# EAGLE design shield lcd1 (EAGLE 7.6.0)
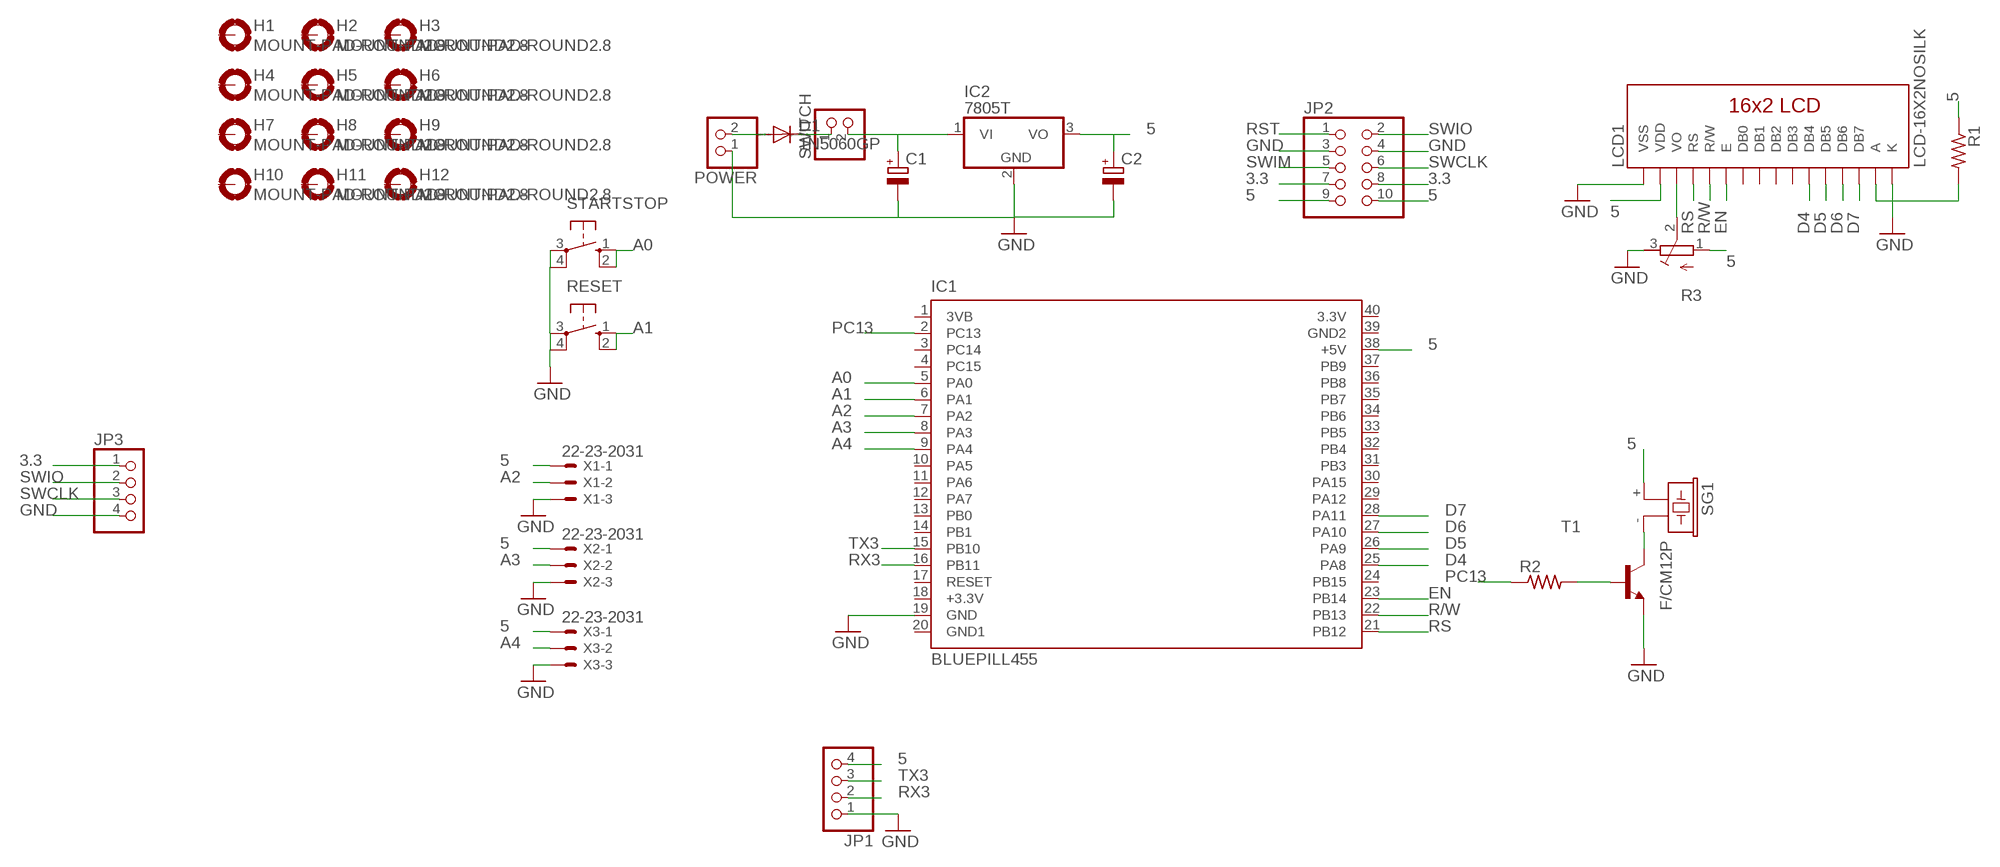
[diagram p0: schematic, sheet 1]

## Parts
C1  CPOL-EUE2.5-7  [E2,5-7]
C2  CPOL-EUE2.5-6  [E2,5-6]
D1  1N5060GP  [DO15-12]
H1  MOUNT-PAD-ROUND2.8  [2,8-PAD]
H2  MOUNT-PAD-ROUND2.8  [2,8-PAD]
H3  MOUNT-PAD-ROUND2.8  [2,8-PAD]
H4  MOUNT-PAD-ROUND2.8  [2,8-PAD]
H5  MOUNT-PAD-ROUND2.8  [2,8-PAD]
H6  MOUNT-PAD-ROUND2.8  [2,8-PAD]
H7  MOUNT-PAD-ROUND2.8  [2,8-PAD]
H8  MOUNT-PAD-ROUND2.8  [2,8-PAD]
H9  MOUNT-PAD-ROUND2.8  [2,8-PAD]
H10  MOUNT-PAD-ROUND2.8  [2,8-PAD]
H11  MOUNT-PAD-ROUND2.8  [2,8-PAD]
H12  MOUNT-PAD-ROUND2.8  [2,8-PAD]
IC1  BLUEPILL455  [DIL40]
IC2  7805T  [TO220H]
JP1  PINHD-1X4  [1X04]
JP2  PINHD-2X5  [2X05]
JP3  PINHD-1X4  [1X04]
LCD1  LCD-16X2NOSILK  [LCD-16X2_NOSILK]
POWER  PINHD-1X2  [1X02]
R1  R-US_0207/10  [0207/10]
R2  R-US_M0805  [M0805]
R3  R-TRIMM3339P  [RTRIM3339P]
RESET  40-XX  [B3F-40XX]
SG1  F/CM12P  [F/CM12P]
STARTSTOP  40-XX  [B3F-40XX]
SWITCH  PINHD-1X2  [1X02]
T1  BF820-NPN-SOT23-BEC  [SOT23-BEC]
X1  22-23-2031  [22-23-2031]
X2  22-23-2031  [22-23-2031]
X3  22-23-2031  [22-23-2031]

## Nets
3.3: JP2.7 JP2.8 JP3.1
5: C2.+ IC1.38(+5V) IC2.3(VO) JP1.4 JP2.9 JP2.10 LCD1.2(VDD) R1.1 R3.1(A) SG1.+ X1.1 X2.1 X3.1
A0: IC1.5(PA0) STARTSTOP.1(S) STARTSTOP.2(S1)
A1: IC1.6(PA1) RESET.1(S) RESET.2(S1)
A2: IC1.7(PA2) X1.2
A3: IC1.8(PA3) X2.2
A4: IC1.9(PA4) X3.2
D4: IC1.25(PA8) LCD1.11(DB4)
D5: IC1.26(PA9) LCD1.12(DB5)
D6: IC1.27(PA10) LCD1.13(DB6)
D7: IC1.28(PA11) LCD1.14(DB7)
EN: IC1.23(PB14) LCD1.6(E)
GND: C1.- C2.- IC1.19(GND) IC2.2(GND) JP1.1 JP2.3 JP2.4 JP3.4 LCD1.1(VSS) LCD1.16(K) POWER.1 R3.3(E) RESET.3(P) RESET.4(P1) STARTSTOP.3(P) STARTSTOP.4(P1) T1.E X1.3 X2.3 X3.3
N$1: LCD1.15(A) R1.2
N$2: R2.2 T1.B
N$9: C1.+ IC2.1(VI) SWITCH.2
N$10: SG1.- T1.C
N$12: LCD1.3(VO) R3.2(S)
N$13: D1.C SWITCH.1
N$14: D1.A POWER.2
PC13: IC1.2(PC13) R2.1
R/W: IC1.22(PB13) LCD1.5(R/W)
RS: IC1.21(PB12) LCD1.4(RS)
RST: JP2.1
RX3: IC1.16(PB11) JP1.2
SWCLK: JP2.6 JP3.3
SWIM: JP2.5
SWIO: JP2.2 JP3.2
TX3: IC1.15(PB10) JP1.3
Unconnected: H1.B2,8(MOUNT) H2.B2,8(MOUNT) H3.B2,8(MOUNT) H4.B2,8(MOUNT) H5.B2,8(MOUNT) H6.B2,8(MOUNT) H7.B2,8(MOUNT) H8.B2,8(MOUNT) H9.B2,8(MOUNT) H10.B2,8(MOUNT) H11.B2,8(MOUNT) H12.B2,8(MOUNT) IC1.1(3VB) IC1.3(PC14) IC1.4(PC15) IC1.10(PA5) IC1.13(PB0) IC1.14(PB1) IC1.17(RESET) IC1.18(+3.3V) IC1.20(GND1) IC1.24(PB15) IC1.29(PA12) IC1.30(PA15) IC1.33(PB5) IC1.34(PB6) IC1.35(PB7) IC1.36(PB8) IC1.37(PB9) IC1.39(GND2) IC1.40(3.3V) LCD1.7(DB0) LCD1.8(DB1) LCD1.9(DB2) LCD1.10(DB3)

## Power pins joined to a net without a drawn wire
PA6: IC1.11(PA6)
PA7: IC1.12(PA7)
PB3: IC1.31(PB3)
PB4: IC1.32(PB4)

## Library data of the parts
C1 C2 = resistor:CPOL-EU: POLARIZED CAPACITOR, European symbol
D1 = diode:1N5060GP: DIODE
H1-H12 = holes:MOUNT-PAD-ROUND: MOUNTING PAD, round
IC1 = STM32BluePill:BLUEPILL: BluePill STM32F108T6 Dev Board Source: http://www.stm32duino.com; 0: x; MF: BluePill; MPN: BluePill; X: 0
IC2 = linear:78*: Positive VOLTAGE REGULATOR Source: http://cache.national.com/ds/LM/LM78L05.pdf http://www.fairchildsemi.com/ds/LM/LM7805.pdf
JP1 JP3 = pinhead:PINHD-1X4: PIN HEADER
JP2 = pinhead:PINHD-2X5: PIN HEADER
LCD1 = SparkFun-Displays:LCD-16X2: Standard text-only 16x2 parallel input LCD Basic 16 character by 2 line display. Typically utilizes the extremely common HD44780 parallel interface chipset SparkFun Products: Basic 16x2 Green Basic 8x2 Green; SF_ID: LCD-00255
POWER SWITCH = pinhead:PINHD-1X2: PIN HEADER
R1 R2 = resistor:R-US_: RESISTOR, American symbol
R3 = resistor:R-TRIMM: Trimm resistor
RESET STARTSTOP = switch-omron:40-XX: OMRON SWITCH; MF: OMRON COMPONENTS USA; MPN: B3F-4000; OC_FARNELL: 176434; OC_NEWARK: 36K3105
SG1 = buzzer:F/CM12P: BUZZER; OC_FARNELL: unknown; OC_NEWARK: unknown
T1 = transistor:*-NPN-: NPN Transistror BF959 corrected 2008.03.06
X1-X3 = con-molex:22-23-2031: .100" (2.54mm) Center Header - 3 Pin; MF: MOLEX; MPN: 22-23-2031; OC_FARNELL: 1462950; OC_NEWARK: 30C0862

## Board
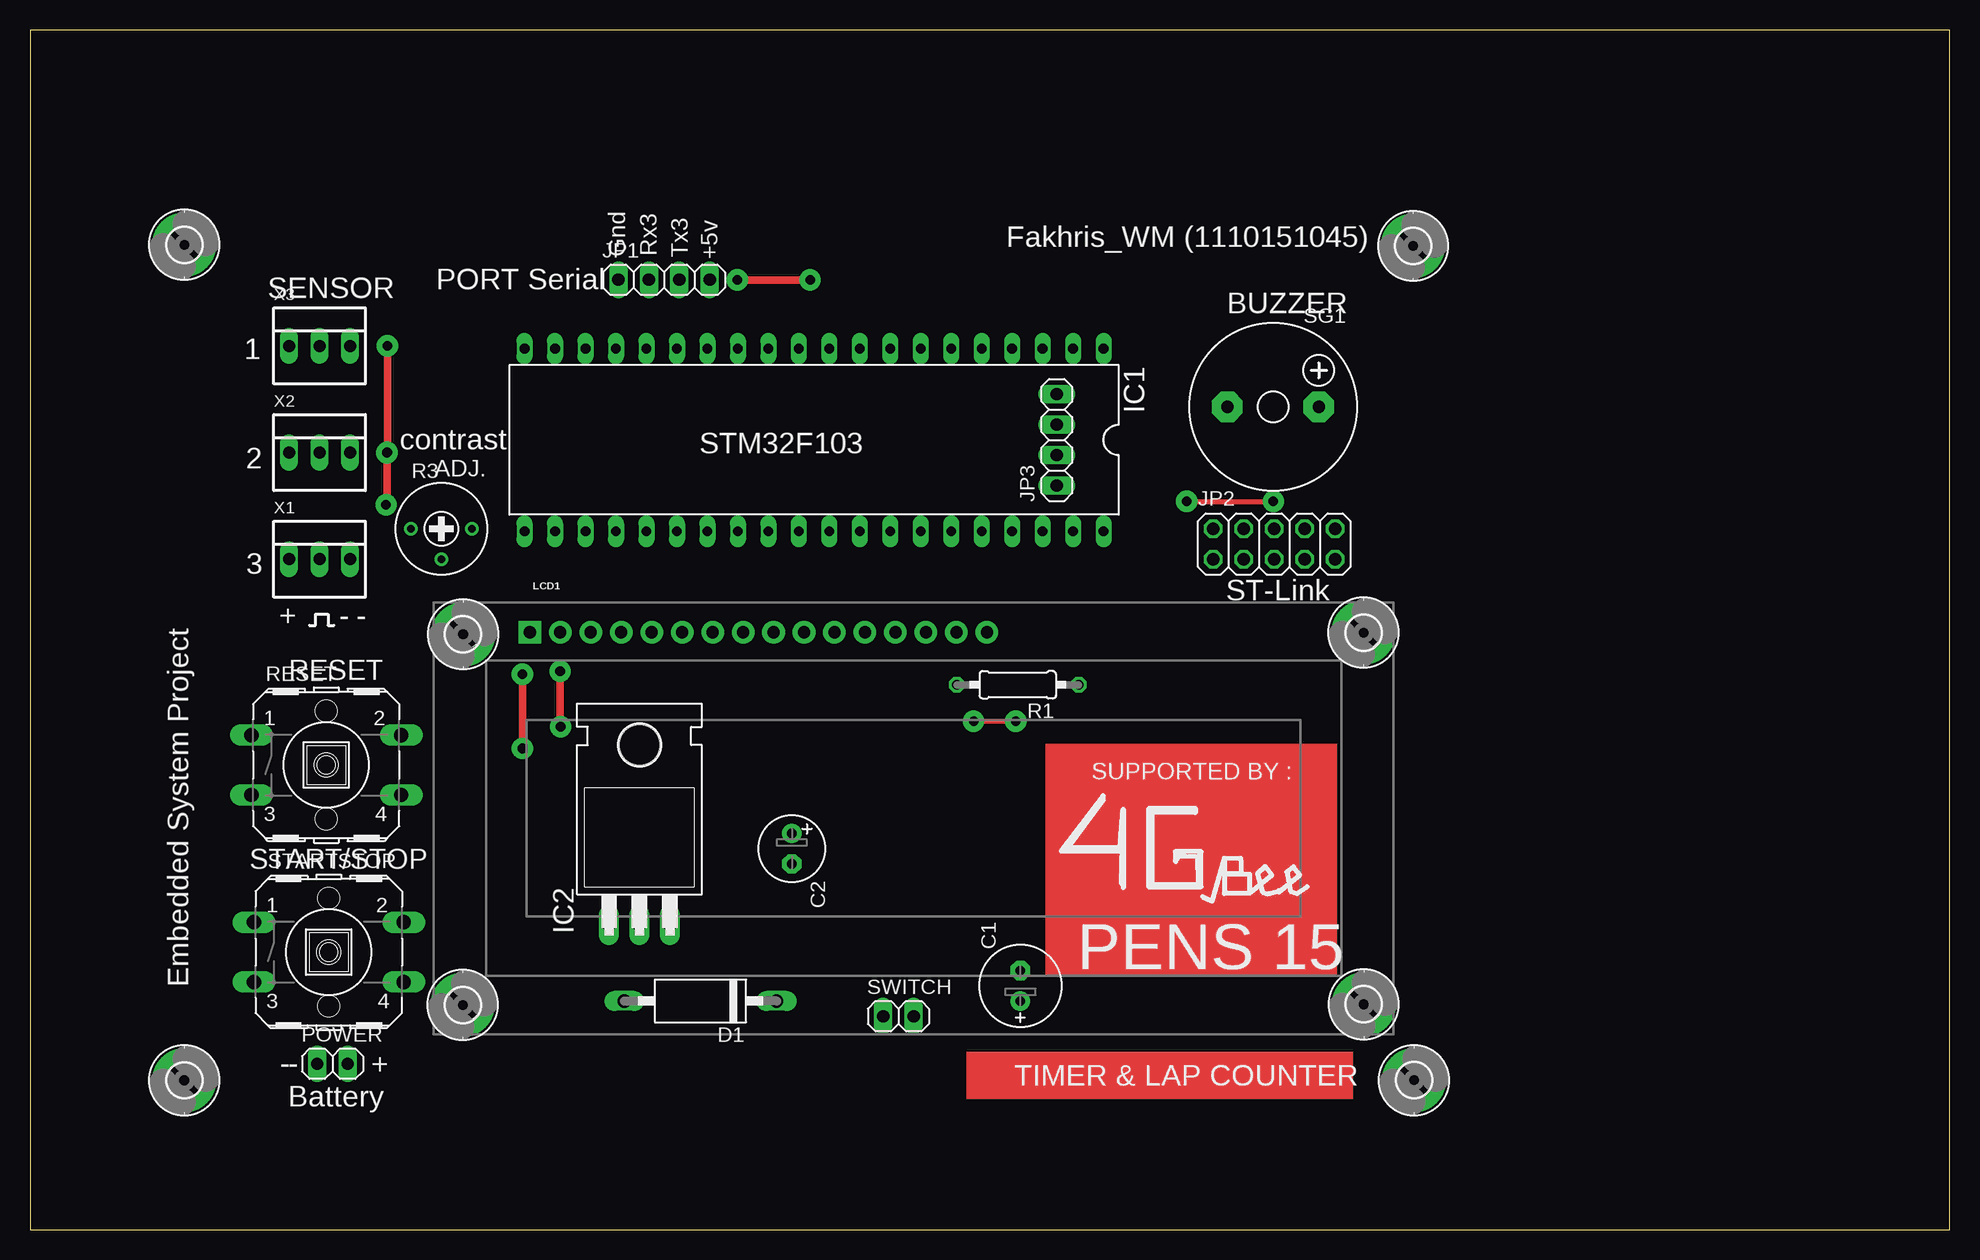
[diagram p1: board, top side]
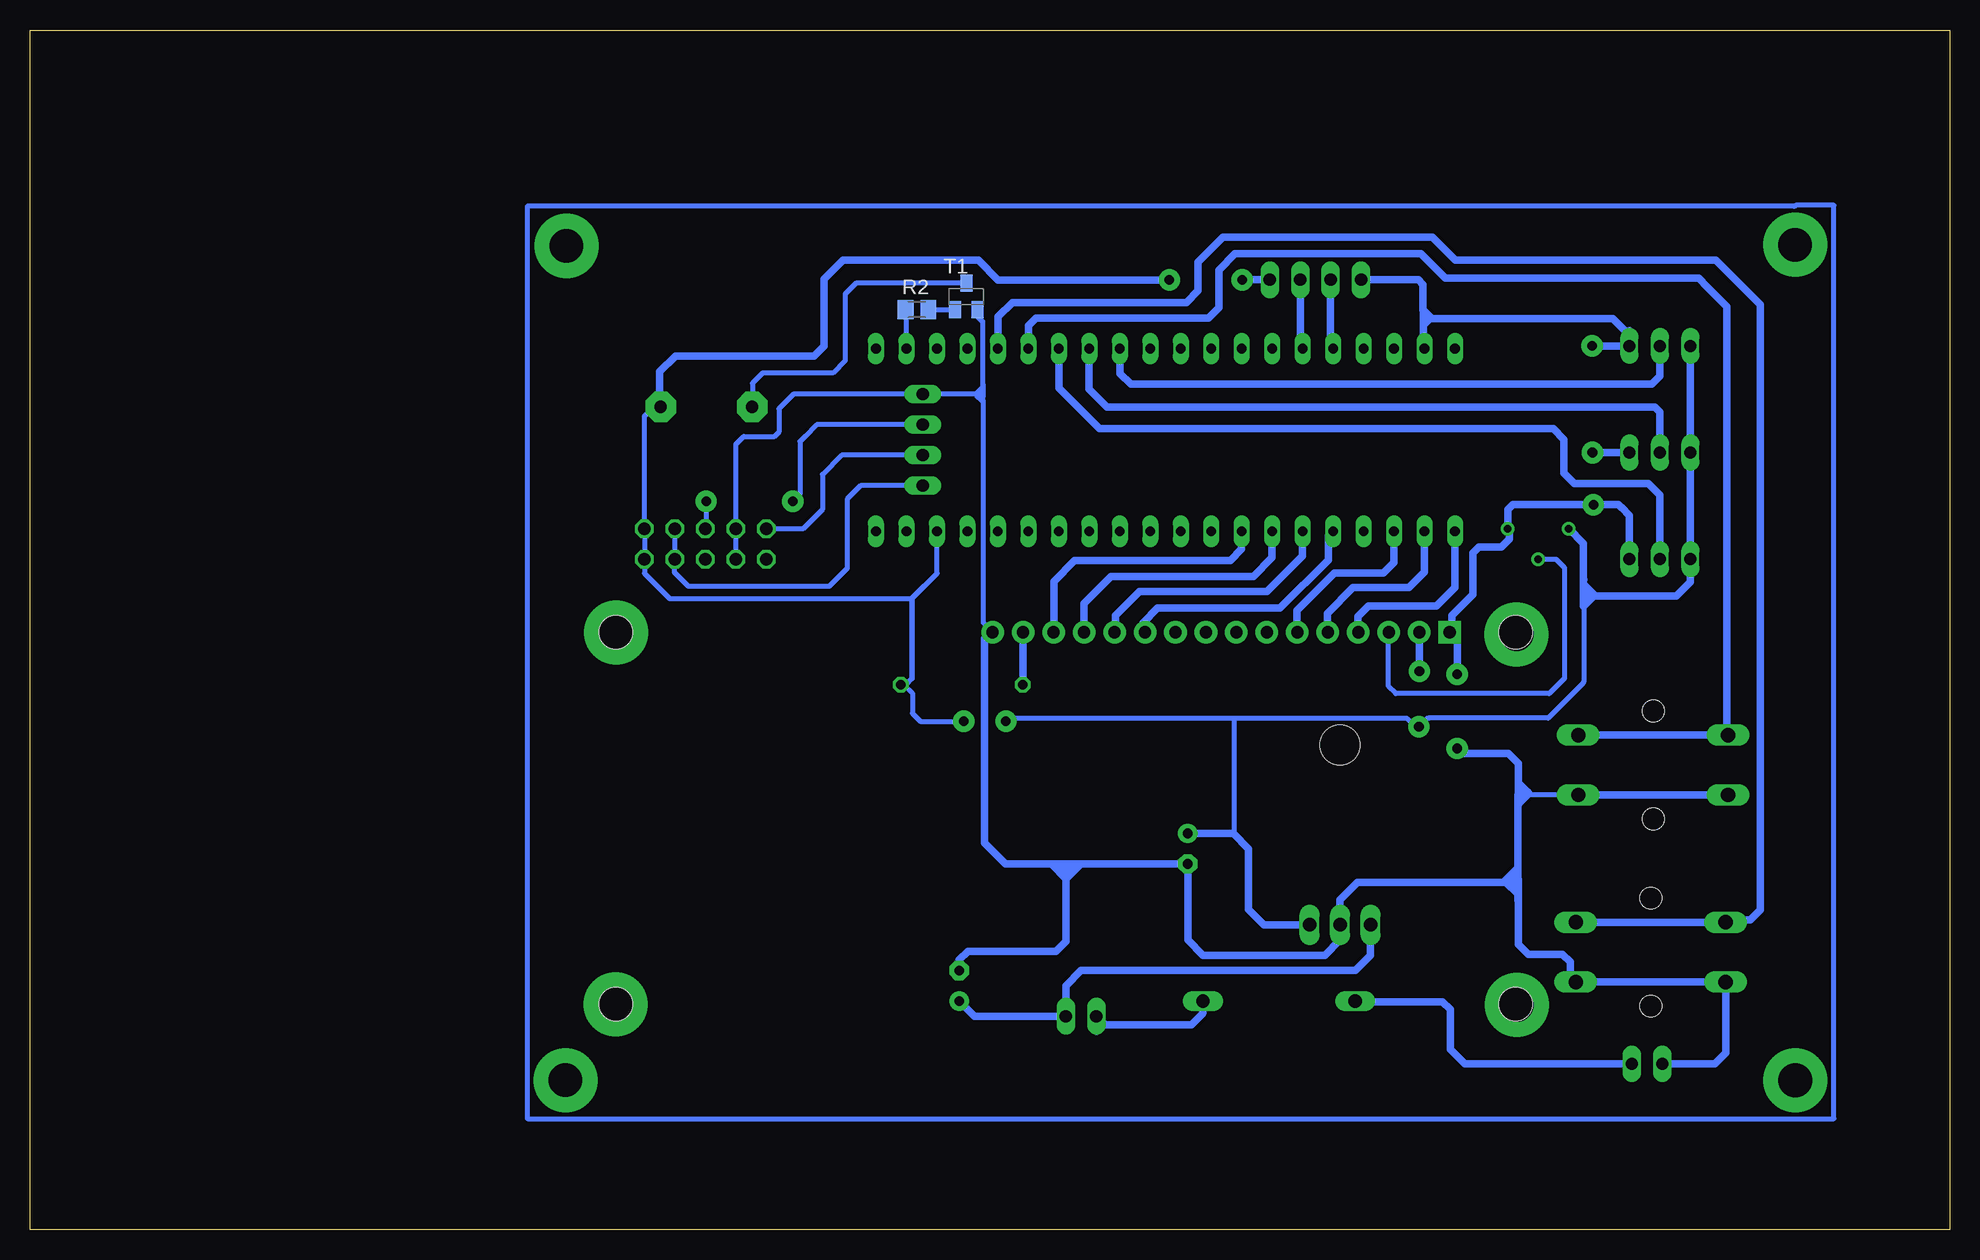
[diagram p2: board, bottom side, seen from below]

Size 160 x 100 mm. Coordinates in mm from the lower left corner, seen from the top.
Outline: 0,0 160,0 160,100 0,100 0,0
Copper layers (1*16): Top 0.035mm / dielectric 1.5mm / Bottom 0.035mm
Design rules "default": minimum track width 10mil, minimum drill 24mil, track to track 8mil, track to pad 8mil, pad to pad 8mil, via to via 8mil, smd to smd 8mil, copper to edge 40mil, drill to drill 8mil, minimum pad ring 10mil, minimum via ring 8mil, stop-mask expansion 4mil, vias tented up to drill 0mil, thermal gap 10mil

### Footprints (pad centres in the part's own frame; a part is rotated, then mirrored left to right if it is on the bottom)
E2,5-7 = drill 0.813 pad 1.6: + -1.27,0 | drill 0.813 pad 1.6 octagon: - 1.27,0
E2,5-6 = drill 0.813 pad 1.6: + -1.27,0 | drill 0.813 pad 1.6 octagon: - 1.27,0
DO15-12 = drill 1.118 long: A 6.35,0; C -6.35,0
2,8-PAD = drill 2.8 pad 5.334: B2,8 0,0
DIL40 = drill 0.813 long: 1 -24.13,-7.62; 2 -21.59,-7.62; 3 -19.05,-7.62; 4 -16.51,-7.62; 5 -13.97,-7.62; 6 -11.43,-7.62; 7 -8.89,-7.62; 8 -6.35,-7.62; 9 -3.81,-7.62; 10 -1.27,-7.62; 11 1.27,-7.62; 12 3.81,-7.62; 13 6.35,-7.62; 14 8.89,-7.62; 15 11.43,-7.62; 16 13.97,-7.62; 17 16.51,-7.62; 18 19.05,-7.62; 19 21.59,-7.62; 20 24.13,-7.62; 21 24.13,7.62; 22 21.59,7.62; 23 19.05,7.62; 24 16.51,7.62; 25 13.97,7.62; 26 11.43,7.62; 27 8.89,7.62; 28 6.35,7.62; 29 3.81,7.62; 30 1.27,7.62; 31 -1.27,7.62; 32 -3.81,7.62; 33 -6.35,7.62; 34 -8.89,7.62; 35 -11.43,7.62; 36 -13.97,7.62; 37 -16.51,7.62; 38 -19.05,7.62; 39 -21.59,7.62; 40 -24.13,7.62
TO220H = drill 1.118 long: 1 -2.54,-10.16; 2 0,-10.16; 3 2.54,-10.16 | hole 3.302: 0,4.826
1X04 = drill 1.016 long: 1 -3.81,0; 2 -1.27,0; 3 1.27,0; 4 3.81,0
2X05 = drill 1.016 octagon: 1 -5.08,-1.27; 2 -5.08,1.27; 3 -2.54,-1.27; 4 -2.54,1.27; 5 0,-1.27; 6 0,1.27; 7 2.54,-1.27; 8 2.54,1.27; 9 5.08,-1.27; 10 5.08,1.27
LCD-16X2_NOSILK = drill 1.016 pad 1.88 square: 1 -32,15.5 | drill 1.016 pad 1.88: 2 -29.46,15.5; 3 -26.92,15.5; 4 -24.38,15.5; 5 -21.84,15.5; 6 -19.3,15.5; 7 -16.76,15.5; 8 -14.22,15.5; 9 -11.68,15.5; 10 -9.14,15.5; 11 -6.6,15.5; 12 -4.06,15.5; 13 -1.52,15.5; 14 1.02,15.5; 15 3.56,15.5; 16 6.1,15.5 | hole 2.8: -37.5,15.5; -37.5,-15.5; 37.5,15.5; 37.5,-15.5
1X02 = drill 1.016 long: 1 -1.27,0; 2 1.27,0
0207/10 = drill 0.813 octagon: 1 -5.08,0; 2 5.08,0
M0805 = smd 1.3 x 1.6: 1 -0.95,0; 2 0.95,0
RTRIM3339P = drill 0.61: 1 -2.54,0; 2 0,-2.54; 3 2.54,0
B3F-40XX = drill 1.194 long: 1 -6.248,2.489; 2 6.248,2.489; 3 -6.248,-2.489; 4 6.248,-2.489 | hole 1.803: 0,-4.496; 0,4.496
F/CM12P = drill 1.016 pad 2.54 octagon: + 3.81,0; - -3.81,0
SOT23-BEC = smd 1 x 1.4: B -0.95,-1.1; C 0,1.1; E 0.95,-1.1
22-23-2031 = drill 1 long: 1 -2.54,0; 2 0,0; 3 2.54,0

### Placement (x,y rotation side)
C1  82.55,20.32 90 top
C2  63.5,31.75 270 top
D1  55.88,19.05 180 top
H1  111.16,49.76 0 top
H2  36.1,49.62 0 top
H3  36.08,18.72 0 top
H4  111.17,18.78 0 top
H5  115.36,12.45 0 top
H6  115.29,82 0 top
H7  12.87,82.09 0 top
H8  12.86,12.44 0 top
H9  not placed on the board
H10  not placed on the board
H11  not placed on the board
H12  not placed on the board
IC1  65.35,65.82 180 top
IC2  50.8,35.56 0 top
JP1  52.85,79.18 0 top
JP2  103.71,57.15 0 top
JP3  85.59,65.83 90 top
LCD1  73.66,34.29 0 top
POWER  25.21,13.82 0 top
R1  82.34,45.41 180 top
R2  86.07,76.69 0 bottom
R3  34.29,58.42 0 top
RESET  24.69,38.72 0 top
SG1  103.62,68.58 0 top
STARTSTOP  24.9,23.13 0 top
SWITCH  72.39,17.78 0 top
T1  81.96,77.78 0 bottom
X1  24.13,55.88 0 top
X2  24.13,64.77 0 top
X3  24.13,73.66 0 top

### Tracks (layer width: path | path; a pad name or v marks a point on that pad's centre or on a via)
3.3
  Bottom 0.406: JP3.1 90.75,62.02 91.89,60.88 91.89,55.11 93.38,53.62 105.11,53.62 106.28,54.78 106.28,55.85 JP2.7 | 106.29,55.83 JP2.7 | JP2.7 JP2.8
5  (via drill 0.8 pad 1.78)
  Top 0.406: v82.17,42.36 78.66,42.36 v78.65,42.37
  Top 0.61: v44.19,46.54 44.19,42.42 v44.23,41.93 | v58.95,79.17 v65.02,79.17 v65.03,79.16
  Bottom 0.254: 58.42,31.75 58.42,31.8 59.62,33
  Bottom 0.406: SG1.+ 108.01,68.58 108.79,67.8 JP2.10 JP2.9 108.79,54.7 106.68,52.6 86.5,52.6 | 86.5,52.6 84.39,54.71 | 84.39,54.71 84.39,58.19 IC1.38 | R1.1 86.99,45.41 86.47,45.93 86.47,52.57 86.5,52.6 | 84.39,54.71 84.4,54.71 86.47,52.63 86.47,45.96 87.03,45.41 87.39,45.41 87.4,45.41 87.14,45.41 86.44,44.72 86.44,43.04 85.77,42.37 v82.17,42.37 v82.17,42.36 | 29.51,52.8 30.47,51.84 30.47,45.75 arc45 30.57,45.52 33.45,42.63 43.4,42.63 arc-45 43.62,42.54 v44.23,41.93 44.41,41.93 arc45 44.64,42.02 45.2,42.59 59.67,42.59 | 59.67,42.59 78.31,42.59 arc-45 78.53,42.49 v78.65,42.37 | 59.62,33 59.62,42.53 59.67,42.59
  Bottom 0.61: X3.1 X2.1 X1.1 21.59,53.98 22.77,52.8 29.51,52.8 30.52,53.81 30.52,57.19 R3.1 31.57,58.6 | LCD1.2 44.2,46.55 v44.19,46.54 | JP1.4 58.94,79.18 v58.95,79.17 | v65.03,79.16 79.32,79.16 80.95,80.8 92.25,80.8 93.8,79.25 93.8,73.67 94.64,72.82 106.2,72.82 107.52,71.5 107.52,68.67 SG1.+ | IC2.3 57.15,25.4 58.42,26.67 58.42,31.75 59.69,33.02 C2.+
A0
  Bottom 0.61: IC1.5 79.3,73.47 79.3,76.09 78.11,77.28 63.62,77.28 62.65,78.25 62.65,80.63 60.55,82.72 43.11,82.72 41.19,80.8 19.46,80.8 15.78,77.12 15.78,26.64 16.62,25.8 19.17,25.8 STARTSTOP.1 STARTSTOP.2
A1
  Bottom 0.61: 76.87,73.53 IC1.6 | 76.89,73.55 IC1.6 | RESET.2 RESET.1 18.56,41.33 18.56,76.96 20.18,78.58 20.91,79.3 42.01,79.3 44.06,81.35 59.55,81.35 60.9,80 60.9,76.86 61.77,75.99 76.15,75.99 76.78,75.36 IC1.6
A2
  Bottom 0.61: X1.2 24.13,61.22 25.1,62.2 31.27,62.2 32.14,63.07 32.14,65.86 33.04,66.75 70.85,66.75 74.23,70.14 IC1.7
A3
  Bottom 0.61: X2.2 24.14,68.16 24.55,68.58 70.23,68.58 71.72,70.07 71.72,73.43 IC1.8
A4
  Bottom 0.61: X3.2 24.13,71.17 24.82,70.48 68.24,70.48 69.13,71.37 69.13,73.41 IC1.9
D4
  Bottom 0.61: LCD1.11 67.23,49.96 67.23,50.58 66.01,51.79 55.81,51.79 51.79,55.81 51.79,57.8 IC1.25
D5
  Bottom 0.61: IC1.26 53.92,56.16 56.9,53.18 67.53,53.18 69.53,51.19 69.53,49.86 LCD1.12
D6
  Bottom 0.61: IC1.27 56.46,56.01 58.03,54.44 69.88,54.44 72.13,52.19 LCD1.13
D7
  Bottom 0.61: IC1.28 59,56.72 59.94,55.79 72.92,55.79 74.67,54.04 74.67,49.8 LCD1.14
EN
  Bottom 0.61: IC1.23 46.3,55.59 47.17,54.72 51.28,54.72 54.38,51.61 54.38,49.81 LCD1.6
GND  (via drill 0.8 pad 1.78)
  Top 0.61: v29.8,73.67 29.8,64.82 v29.77,64.79 | v29.76,64.75 29.76,60.65 v29.68,60.42 | v41.05,40.1 41.05,46.26 v41.03,46.28
  Bottom 0.406: RESET.4 35.07,36.23 35.07,36.35 | T1.E 81.01,76.12 80.59,75.7 80.59,70.17 81.13,69.63 | 81.13,69.63 JP3.4 96.37,69.64 97.57,68.43 97.54,68.4 97.54,66.53 97.95,66.12 100.51,66.12 101.17,65.47 101.17,60.32 101.17,60.31 JP2.4 JP2.3 | 81.13,69.63 81.13,69.58 80.64,69.09 80.56,69.02 80.56,50.59 LCD1.16
  Bottom 0.61: 26.67,74.93 X3.3 | 73.63,29.24 73.66,29.21 73.66,24.01 74.46,23.21 81.83,23.21 82.57,22.47 82.57,21.61 C1.- | 73.63,29.24 72.39,30.48 C2.- 63.5,24.13 62.23,22.86 52.07,22.86 50.8,24.13 IC2.2 50.8,27.48 49.34,28.95 37.18,28.95 | LCD1.1 | X3.3 26.67,74.55 28.08,75.95 43.3,75.95 43.84,75.41 | 43.84,73.51 IC1.19 43.84,73.51 43.84,75.41 | X1.3 26.67,59.51 27.33,60.17 27.34,60.17 27.59,60.42 v29.68,60.42 36.4,60.42 36.8,60.02 36.8,58.45 R3.3 36.7,58.29 36.7,57.55 37.35,56.9 39.21,56.9 39.74,56.38 39.74,52.93 41.49,51.17 41.49,49.95 LCD1.1 | LCD1.1 41.76,49.69 41.67,49.69 41.03,49.05 v41.03,46.28 | 37.18,28.95 35.99,30.13 35.99,35.43 35.07,36.35 35.93,37.22 35.93,38.87 36.77,39.7 40.62,39.7 40.63,39.68 v41.05,40.1 | 37.18,28.95 36.96,28.95 35.95,27.93 35.95,23.76 35.12,22.93 32.26,22.93 31.62,22.3 31.62,21.11 STARTSTOP.4 | 31.72,20.78 STARTSTOP.4 | 23.88,13.88 POWER.1 19.58,13.83 18.66,14.75 18.66,20.1 | RESET.3 RESET.4 | STARTSTOP.3 18.66,20.1 | STARTSTOP.4 19.2,20.64 18.66,20.1 | LCD1.16 79.93,49.79 80.44,49.28 80.44,32.23 79.17,30.96 78.69,30.48 74.87,30.48 73.63,29.24 | X3.3 29.78,73.66 v29.8,73.67 | v29.77,64.79 26.69,64.79 X2.3 29.74,64.77 v29.76,64.75 | 43.84,75.41 43.84,75.42 43.31,75.95 43.31,76.09 43.89,76.67 43.89,78.79 44.27,79.17 JP1.1
N$1
  Bottom 0.61: LCD1.15 77.22,45.45 R1.2
N$2
  Bottom 0.406: R2.2 T1.B
N$3
  Bottom 0.61: 35.98,30.61 arc90 35.98,30.61 35.98,27.44 arc-90 35.95,27.47 35.95,29.19 36.28,29.19 arc-90 36.32,29.15 36.32,28.97
N$4
  Bottom 0.61: 35.16,36.46 35.66,36.46 arc-90 35.97,36.14 35.97,35.39 arc-90 35.94,35.42 35.94,37.2
N$5
  Bottom 0.61: 71.82,30.47 75.11,30.47 arc90 75.13,30.5 74.02,30.5 arc90 73.71,30.18 73.71,29.64 arc90 74.01,29.95 74.01,30.05 73.52,30.05 arc-90 73.44,30.13
N$6
  Bottom 0.61: 30.49,54.17 arc-90 30.5,54.16 30.5,51.97
N$7
  Bottom 0.61: 29.7,52.76 30,52.76 arc90 30.26,53.02 arc-90 30.32,52.97 30.32,52.53
N$8
  Bottom 0.406: 118.53,9.25 9.64,9.25 9.64,85.38 12.82,85.38 12.85,85.32
N$9
  Bottom 0.61: C1.+ 81.28,17.78 SWITCH.2 73.66,20.32 72.39,21.59 49.53,21.59 48.26,22.86 IC2.1
N$10
  Bottom 0.406: T1.C 91.15,78.88 92.04,77.99 92.04,72.45 93.08,71.41 98.93,71.41 99.79,70.55 99.79,68.6 SG1.-
N$12
  Bottom 0.406: R3.2 34.27,55.86 32.78,55.86 32.09,55.17 32.09,45.95 33.36,44.67 46.15,44.67 46.75,45.28 46.75,49.76 arc45 LCD1.3
  Bottom 0.61: 34.17,56 R3.2
N$13
  Bottom 0.61: 71.12,16.51 SWITCH.1 70.51,17.17 arc-45 70.29,17.08 63.17,17.08 62.32,17.93 arc-45 62.23,18.15 D1.C
N$14
  Bottom 0.61: POWER.2 40.39,13.81 41.6,15.03 41.6,18.34 42.26,19 49.48,19 D1.A
N$15
  Bottom 0.406: 80.57,70.42 80.56,70.42 80.56,69.48 | 80.56,69.09 80.56,69.48 | 80.56,69.48 80.7,69.62
N$16
  Bottom 0.406: 43.86,75.34 43.86,76.63 43.95,76.72 43.95,76.66 43.98,76.63
N$17
  Bottom 0.406: 43.9,76.76 43.9,76.69 43.97,76.61 43.97,75.48 43.92,75.42
N$18
  Bottom 0.406: 12.97,85.3 118.56,85.3 118.56,9.38
PC13
  Bottom 0.406: IC1.2 86.94,76.61 R2.1
R/W
  Bottom 0.61: IC1.22 43.76,54.82 45.08,53.5 49.73,53.5 51.87,51.36 51.87,49.84 LCD1.5
RS
  Bottom 0.61: IC1.21 41.22,53.54 42.79,51.97 48.42,51.97 49.29,51.09 49.29,49.8 LCD1.4
RX3
  Bottom 0.61: JP1.2 51.58,73.64 IC1.16
SWCLK  (via drill 0.8 pad 1.78)
  Top 0.406: v96.42,60.7 103.5,60.7 v103.64,60.71
  Bottom 0.406: JP3.3 94.43,67.09 95.41,66.11 | v103.64,60.71 103.64,58.48 JP2.6 | 95.41,66.11 | 95.41,66.11 95.83,65.69 95.83,61.29 v96.42,60.7
SWIO
  Bottom 0.406: JP3.2 92.35,64.56 93.95,62.95 93.95,60.02 95.58,58.4 98.6,58.4 JP2.2
TX3
  Bottom 0.61: JP1.3 54.12,73.64 IC1.15
(copper drawn outside any net)
  shapes: Top area x2

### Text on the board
tPlace: Fakhris_WM (1110151045) | Gnd | Rx3 | Tx3 | +5v | SENSOR | PORT Serial | BUZZER | 1 | contrast | STM32F103 | 2 | ADJ. | 3 | ST-Link | + - | - | RESET | SUPPORTED BY : | START/STOP | PENS 15 | Embedded System Project | - | - | + | TIMER & LAP COUNTER | Battery

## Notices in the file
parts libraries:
SparkFun-Displays: Licensing: Creative Commons ShareAlike 4.0 International - https://creativecommons.org/licenses/by-sa/4.0
